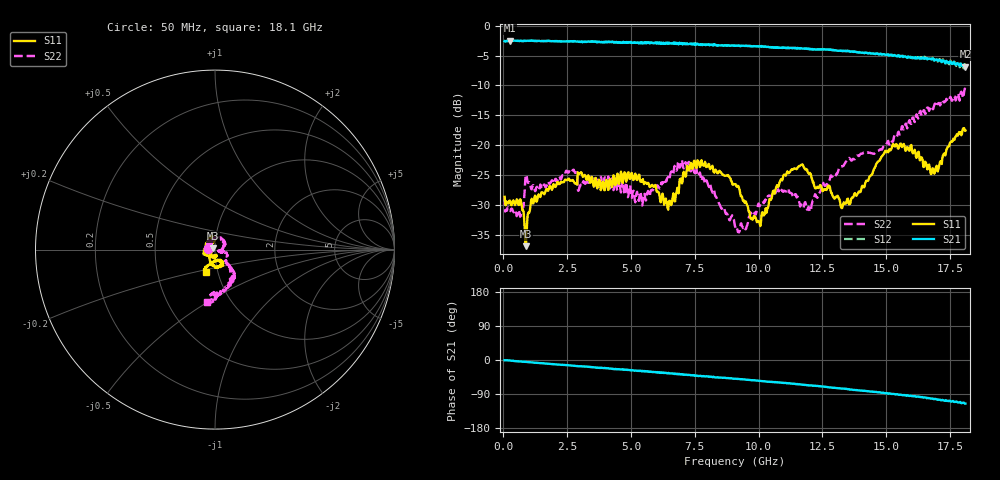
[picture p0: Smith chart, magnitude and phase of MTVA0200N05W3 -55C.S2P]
! Network Analyzer HP8720D.06.14 Serial No. US36140669
! 17 Jan 2005  13:49:12
! Frequency  S11  S21  S12  S22
# HZ  S  DB R 50
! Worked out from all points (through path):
!   801 points, 50 MHz to 18.1 GHz, reference 50 ohm
!   highest |S21| = -2.48 dB at 253.1 MHz (marker M1); lowest = -6.9 dB at 18.1 GHz (marker M2)
!   group delay of S21, straight-line fit = 16.8 ps
!   lowest |S11| = -36.9 dB at 884.8 MHz (marker M3), VSWR 1.03, Z = 48.8 + j0.657 ohm
!   |S11| at or under -10 dB: start of sweep to end of sweep
!   |S22| runs from -34.6 to -10.5 dB; largest |S21 - S12| = 0.026
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5e7  -28.64 -178.8  -2.59 -0.8  -2.58 -1.0  -28.69 175.5
2.530625e8  -29.26 164.7  -2.48 -1.2  -2.51 -1.7  -30.93 172.3
7.043125e8  -29.81 132.7  -2.55 -4.3  -2.54 -4.4  -31.50 179.3
8.848125e8  -36.90 151.9  -2.55 -4.9  -2.51 -5.3  -25.01 175.5
1.178125e9  -29.75 148.5  -2.53 -7.1  -2.55 -7.3  -26.69 143.4
2.66725e9  -25.89 114.8  -2.60 -14.6  -2.60 -15.1  -24.45 121.0
3.073375e9  -24.68 107.6  -2.66 -16.9  -2.62 -17.2  -26.79 146.8
5.510125e9  -26.51 126.0  -2.94 -29.9  -2.91 -30.2  -28.45 129.1
6.074188e9  -27.80 146.4  -2.97 -33.3  -2.96 -33.3  -26.96 119.4
6.525438e9  -29.30 144.4  -2.96 -35.3  -2.93 -35.0  -25.20 104.6
7.202312e9  -23.41 109.6  -2.95 -39.4  -3.03 -39.7  -23.96 51.0
7.834062e9  -23.39 109.3  -3.15 -42.4  -3.11 -43.3  -25.45 19.7
9.075e9  -26.52 177.7  -3.37 -49.4  -3.34 -49.9  -33.56 -23.1
1.000006e10  -32.70 -167.6  -3.46 -54.9  -3.46 -55.1  -29.75 -20.8
1.10605e10  -25.11 174.9  -3.73 -60.9  -3.74 -61.3  -27.72 -20.4
1.166969e10  -23.27 -159.4  -3.75 -64.9  -3.76 -65.3  -29.92 -24.2
1.209838e10  -25.71 -139.5  -3.89 -67.6  -3.92 -68.0  -29.61 -11.8
1.331675e10  -29.74 -80.3  -4.22 -75.6  -4.19 -75.8  -23.47 -16.6
1.509919e10  -20.93 -93.2  -4.99 -88.7  -4.85 -89.3  -19.75 -50.5
1.591144e10  -20.91 -66.1  -5.29 -94.8  -5.27 -94.2  -15.79 -54.1
1.68365e10  -23.90 -83.8  -5.54 -102.5  -5.50 -104.2  -13.98 -66.0
1.81e10  -17.56 -111.1  -6.87 -115.1  -6.62 -115.5  -10.63 -98.6
